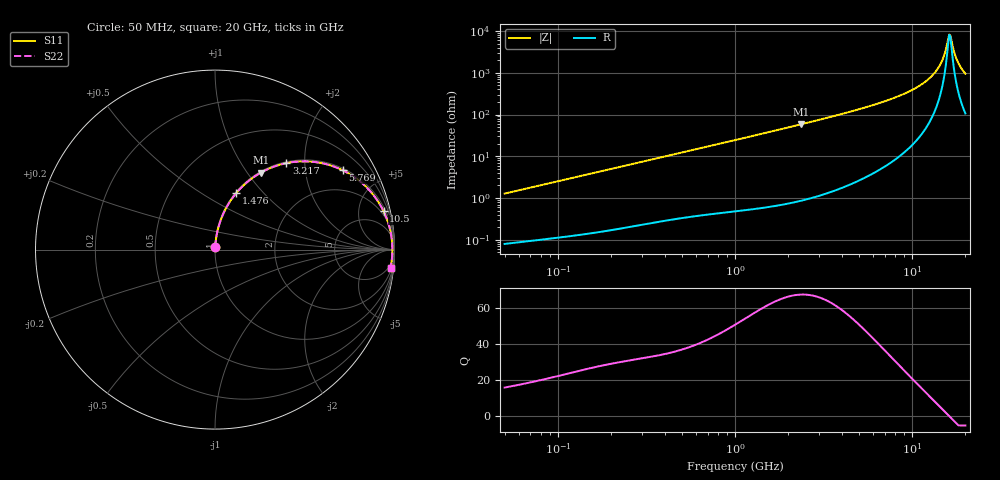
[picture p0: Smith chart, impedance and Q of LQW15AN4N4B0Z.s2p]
!Murata Part Number: LQW15AN4N4B0Z
!These Parameters are Measured in Series Mode Connection
!  o--[Z]--o
!Port1  Port2
!  o-------o
!Freq. Start=50[MHz] Stop=20[GHz], 401[Steps]
# Hz S RI R 50
!Freq.(Hz) S11(Real) S11(Imag) S21(Real) S21(Imag) S12(Real) S12(Imag) S22(Real) S22(Imag)
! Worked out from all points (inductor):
!   401 points, 50 MHz to 20 GHz, reference 50 ohm
!   read as one part in series: L = 4.04 nH near 51.52 MHz
!   highest Q = 67.6 at 2.349 GHz (marker M1), where L = 3.93 nH
!   self-resonance near 16.22 GHz
!   S11 on the Smith chart (normalised r, x): 50 MHz: 1.00, +0.03; 1.476 GHz: 1.01, +0.72; 3.217 GHz: 1.02, +1.62; 5.769 GHz: 1.07, +3.19; 10.5 GHz: 1.46, +8.65; 20 GHz: 3, -19
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5e7  0.00096 0.0128  0.999 -0.0128  0.999 -0.0128  0.00096 0.0128
1.364002e8  0.00249 0.0341  0.9975 -0.0341  0.9975 -0.0341  0.00249 0.0341
3.721004e8  0.011 0.0905  0.989 -0.0905  0.989 -0.0905  0.011 0.0905
1e9  0.0601 0.228  0.9399 -0.228  0.9399 -0.228  0.0601 0.228
1.476162e9  0.119 0.3157  0.881 -0.3157  0.881 -0.3157  0.119 0.3157
2.348516e9  0.2549 0.4284  0.7451 -0.4284  0.7451 -0.4284  0.2549 0.4284
2.728004e9  0.3178 0.4582  0.6822 -0.4582  0.6822 -0.4582  0.3178 0.4582
3.216634e9  0.3971 0.4816  0.6029 -0.4816  0.6029 -0.4816  0.3971 0.4816
4.34015e9  0.5592 0.4877  0.4408 -0.4877  0.4408 -0.4877  0.5592 0.4877
5.769027e9  0.7131 0.4414  0.2869 -0.4414  0.2869 -0.4414  0.7131 0.4414
7.442007e9  0.8304 0.3609  0.1696 -0.3609  0.1696 -0.3609  0.8304 0.3609
1.050288e10  0.9392 0.2138  0.0608 -0.2138  0.0608 -0.2138  0.9392 0.2138
1.238412e10  0.9692 0.1353  0.0308 -0.1353  0.0308 -0.1353  0.9692 0.1353
1.396067e10  0.9822 0.0767  0.0178 -0.0767  0.0178 -0.0767  0.9822 0.0767
1.482269e10  0.986 0.0471  0.014 -0.0471  0.014 -0.0471  0.986 0.0471
1.597544e10  0.9882 0.00995  0.0118 -0.00995  0.0118 -0.00995  0.9882 0.00995
1.621653e10  0.9883 0.00252  0.0117 -0.00252  0.0117 -0.00252  0.9883 0.00252
1.670968e10  0.9882 -0.0123  0.0118 0.0123  0.0118 0.0123  0.9882 -0.0123
1.747767e10  0.9871 -0.0346  0.0129 0.0346  0.0129 0.0346  0.9871 -0.0346
1.828096e10  0.9851 -0.0569  0.0149 0.0569  0.0149 0.0569  0.9851 -0.0569
1.940974e10  0.9808 -0.0864  0.0192 0.0864  0.0192 0.0864  0.9808 -0.0864
2e10  0.9779 -0.1012  0.0221 0.1012  0.0221 0.1012  0.9779 -0.1012
